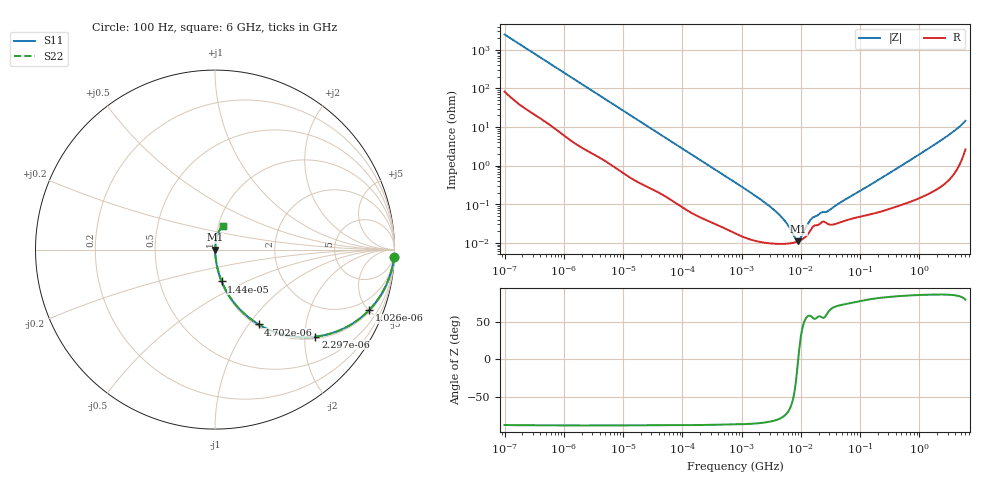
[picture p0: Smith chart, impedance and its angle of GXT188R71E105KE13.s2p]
!Murata Part Number: GXT188R71E105KE13
!These Parameters are Measured in Series Mode Connection
!Data Generated on Jan 08, 2026
!  o--ll--o
!Port1  Port2
!  o------o
!Operation Temp=25[degC], DC Bias Voltage=0[V]
!Freq. Start=100[Hz] Stop=6[GHz] 401[Steps]
# Hz S RI R 50
!Freq.(Hz) S11(Real) S11(Imag) S21(Real) S21(Imag) S12(Real) S12(Imag) S22(Real) S22(Imag)
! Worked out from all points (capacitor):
!   401 points, 100 Hz to 6 GHz, reference 50 ohm
!   read as one part in series: C = 637 nF near 109 Hz
!   lowest |Z| = 11 mohm at 9.09 MHz (marker M1)
!   series resonance near 9.049 MHz, so ESL is about 490 pH
!   S11 on the Smith chart (normalised r, x): 100 Hz: 3, -50; 1.026 kHz: 1.12, -5.01; 2.297 kHz: 1.05, -2.26; 4.702 kHz: 1.03, -1.12; 14.4 kHz: 1.01, -0.37; 6 GHz: 1.05, +0.28
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100  0.9971 -0.04  0.00293 0.04  0.00293 0.04  0.9971 -0.04
350  0.9777 -0.135  0.0223 0.135  0.0223 0.135  0.9777 -0.135
1026  0.857 -0.3387  0.143 0.3387  0.143 0.3387  0.857 -0.3387
2008  0.6221 -0.4737  0.3779 0.4737  0.3779 0.4737  0.6221 -0.4737
2297  0.5595 -0.4852  0.4405 0.4852  0.4405 0.4852  0.5595 -0.4852
4702  0.243 -0.4167  0.757 0.4167  0.757 0.4167  0.243 -0.4167
7695  0.1117 -0.303  0.8883 0.303  0.8883 0.303  0.1117 -0.303
14402  0.0372 -0.1776  0.9628 0.1776  0.9628 0.1776  0.0372 -0.1776
40335  0.00645 -0.0667  0.9936 0.0667  0.9936 0.0667  0.00645 -0.0667
774597  0.000189 -0.00368  0.9998 0.00368  0.9998 0.00368  0.000189 -0.00368
2169299  0.000105 -0.00127  0.9999 0.00127  0.9999 0.00127  0.000105 -0.00127
3882480  9.42e-05 -0.000618  0.9999 0.000618  0.9999 0.000618  9.42e-05 -0.000618
5809218  9.45e-05 -0.0003  0.9999 0.0003  0.9999 0.0003  9.45e-05 -0.0003
8311524  0.000104 -5.66e-05  0.9999 5.66e-05  0.9999 5.66e-05  0.000104 -5.66e-05
9090158  0.00011 3.1e-06  0.9999 -3.1e-06  0.9999 -3.1e-06  0.00011 3.1e-06
9941735  0.000117 6.34e-05  0.9999 -6.34e-05  0.9999 -6.34e-05  0.000117 6.34e-05
1.360128e7  0.000178 0.000286  0.9998 -0.000286  0.9998 -0.000286  0.000178 0.000286
1.555665e7  0.000244 0.000363  0.9998 -0.000363  0.9998 -0.000363  0.000244 0.000363
2.911731e7  0.000302 0.000598  0.9997 -0.000598  0.9997 -0.000598  0.000302 0.000598
3.124326e8  0.000788 0.00631  0.9992 -0.00631  0.9992 -0.00631  0.000788 0.00631
2.34314e9  0.00489 0.045  0.9951 -0.045  0.9951 -0.045  0.00489 0.045
6e9  0.0437 0.1318  0.9563 -0.1318  0.9563 -0.1318  0.0437 0.1318
